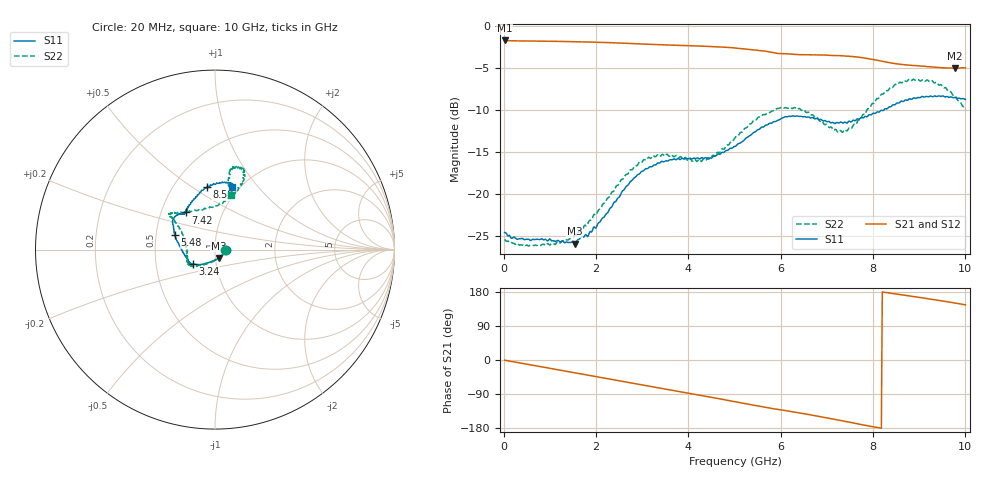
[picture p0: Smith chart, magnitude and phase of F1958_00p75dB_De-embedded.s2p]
! Integrated Device Technology
! Corporate Headquarters
! 6024 Silver Creek Valley Road
! San Jose, CA 95138  USA
! Phone:  1-408-284-8200
! Toll Free:  1-800-223-1366
! Webpage:  http://www.idt.com/
! Timing and RF Division
! 515 Groton Road, Suite 102
! Westford, MA 01886-6024
! Device:  F1958
! Description: 7-bit 0.25 dB Digital Step Attenuator
! Frequency:  0.001 -  6.000 GHz
! Package:  4x4 mm Thin QFN Plastic Package: 24 pin
! Ports:  2 RF, 12 DC
!  Pin  1  = D0
!  Pin  2  = VDD
!  Pin  3  = VMODE
!  Pin  4  = GND
!  Pin  5  = RF1  =  Port 1
!  Pin  6  = GND
!  Pin  7  = GND
!  Pin  8  = GND
!  Pin  9  = GND
!  Pin 10  = GND
!  Pin 11  = GND
!  Pin 12  = GND
!  Pin 13  = GND
!  Pin 14  = RF2  =  Port 2
!  Pin 15  = GND
!  Pin 16  = LE
!  Pin 17  = CLK
!  Pin 18  = DATA
!  Pin 19  = D6
!  Pin 20  = D5
!  Pin 21  = D4
!  Pin 22  = D3
!  Pin 23  = D2
!  Pin 24  = D1
! State:  3
! Atten State:  0.75 dB
! Voltage:  +3.30 Volts
! Current:  0.258 mA
! Data:  The device was measured on a F1958 evaluation board which has
!  individual transmission lines to the RF pins.  Data was collected
!  using a calibrated network analyzer.  The evaluation board was
!  de-embedded using Automatic Fixture Removal (AFR).
!  The reference plane is the edge of the package pin.
! Misc:
!  Action Tracker AT0419
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# GHz S dB R 50
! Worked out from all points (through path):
!   500 points, 20 MHz to 10 GHz, reference 50 ohm
!   highest |S21| = -1.75 dB at 20 MHz (marker M1); lowest = -5.1 dB at 9.78 GHz (marker M2)
!   group delay of S21, straight-line fit = 60.2 ps
!   lowest |S11| = -26.0 dB at 1.54 GHz (marker M3), VSWR 1.11, Z = 51.9 - j4.78 ohm
!   |S11| at or under -10 dB: start of sweep to 8.24 GHz
!   |S22| runs from -26.3 to -6.4 dB; largest |S21 - S12| = 0.0021
!   S11 on the Smith chart (normalised r, x): 20 MHz: 1.12, -0.01; 3.24 GHz: 0.77, -0.13; 5.48 GHz: 0.63, +0.11; 7.42 GHz: 0.67, +0.30; 8.58 GHz: 0.73, +0.57; 10 GHz: 0.92, +0.75
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0.02  -24.63 -2.5  -1.75 -0.6  -1.75 -0.6  -25.46 -3.0
0.3  -25.45 -7.9  -1.80 -6.7  -1.81 -6.7  -25.94 -12.0
0.76  -25.47 -19.2  -1.83 -16.7  -1.83 -16.6  -26.10 -27.7
1.54  -25.95 -65.8  -1.90 -33.7  -1.90 -33.7  -24.94 -81.0
1.7  -25.14 -76.9  -1.92 -37.2  -1.92 -37.2  -24.35 -92.2
2.02  -23.83 -100.7  -1.97 -44.2  -1.96 -44.2  -22.36 -110.6
2.72  -18.77 -134.3  -2.10 -59.6  -2.09 -59.6  -17.37 -137.5
3.24  -16.65 -147.0  -2.24 -71.0  -2.24 -71.1  -15.48 -147.9
3.36  -16.35 -148.3  -2.26 -73.6  -2.27 -73.7  -15.48 -149.4
4.32  -15.81 -160.8  -2.43 -94.6  -2.45 -94.6  -15.88 178.9
5.02  -14.35 176.9  -2.65 -110.3  -2.66 -110.3  -13.26 151.6
5.48  -12.47 160.2  -2.92 -120.5  -2.93 -120.5  -11.13 144.3
6  -11.10 148.0  -3.31 -131.3  -3.32 -131.3  -9.75 142.4
6.68  -10.94 135.4  -3.47 -145.5  -3.49 -145.4  -10.62 135.2
7.2  -11.57 130.4  -3.56 -157.3  -3.57 -157.2  -12.38 110.7
7.42  -11.58 128.4  -3.62 -162.6  -3.63 -162.5  -12.51 95.3
7.92  -10.59 117.4  -3.94 -174.4  -3.94 -174.4  -9.88 72.2
8.34  -9.70 105.4  -4.38 177.0  -4.38 176.9  -7.62 67.4
8.58  -9.13 97.2  -4.59 172.7  -4.59 172.8  -6.72 69.5
9.26  -8.40 80.2  -4.90 160.2  -4.91 160.2  -6.55 77.1
9.78  -8.53 74.6  -5.06 150.4  -5.08 150.4  -8.38 78.0
10  -8.78 74.7  -5.01 145.4  -5.04 145.5  -9.96 73.4
